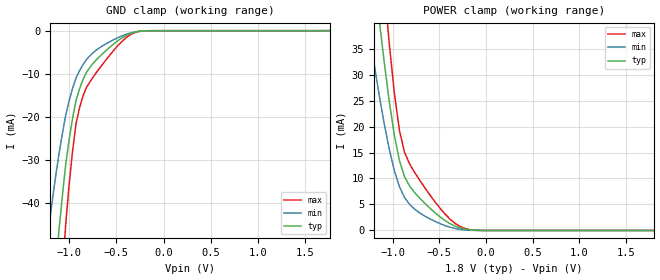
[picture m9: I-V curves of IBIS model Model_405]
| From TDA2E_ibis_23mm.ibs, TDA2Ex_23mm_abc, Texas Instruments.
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| Model based on original model for CAMERARX_CORE
|   Sub model CAMERARX_CORE_PUPD0
[model]   Model_405
|[Description]  [1.8V-INPUT-X-X]
|   , ,
|[Input Load]
|[Output Drive]
|Voltage   1.8V
|Mode   INPUT
Model_type   Input
Polarity   Non-Inverting
Vinl =  0.63
Vinh =  1.17
C_comp   1.75p   1.5p   2p
[Model Spec]
Vinl   0.63   0.567   0.6615
Vinh   1.17   1.053   1.2285
[Temperature Range]   25   125   -40
[Voltage Range]   1.8   1.62   1.92
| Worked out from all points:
|   GND clamp passes 1 mA (typ) near -0.39 V on its own axis
|   POWER clamp passes 1 mA (typ) near -0.35 V on its own axis
[POWER_clamp]
-1.8V     156.8mA    109.4mA    217.7mA
-1.255V   58.58mA    38.5mA     83.58mA
-1.127V   37.93mA    24.29mA    54.73mA
-1.055V   27.33mA    17.27mA    39.59mA
-981.8mV  18.3mA     11.5mA     26.4mA
-927.3mV  13.42mA    8.419mA    19.22mA
-872.7mV  10.36mA    6.348mA    15.04mA
-818.2mV  8.551mA    5.012mA    12.79mA
-654.5mV  5.218mA    2.76mA     8.209mA
-381.8mV  1.281mA    612uA      2.13mA
-163.6mV  106uA      34.63uA    142.1uA
1.8V      2.655uA    1.447uA    5.48uA
[GND_clamp]
-1.8V     -252.1mA   -161mA     -379.9mA
-1.218V   -74.99mA   -46.16mA   -113.7mA
-1.109V   -46.67mA   -28.87mA   -69.57mA
-1.036V   -31.06mA   -19.64mA   -44.89mA
-963.6mV  -20.33mA   -13.39mA   -27.93mA
-927.3mV  -16.23mA   -11mA      -21.58mA
-854.5mV  -11.42mA   -7.916mA   -15.25mA
-818.2mV  -9.733mA   -6.736mA   -13.26mA
-636.4mV  -5.156mA   -3.402mA   -7.535mA
-418.2mV  -1.379mA   -1.021mA   -2.048mA
-272.7mV  -182.6uA   -178.1uA   -212.2uA
1.764V    1.345uA    26.47uA    2.07uA
